TYPE ST_Control_UINT_TO_BIT :
STRUCT
	Enable_latch_C									:	BIT;
	Enable_latch_extern_on_positive_edge			:	BIT;
	Set_counter										:	BIT;
	Enable_latch_extern_on_negative_edge			:	BIT;
	{attribute 'hide'}
	reserve_b5										:	BIT;
	{attribute 'hide'}
	reserve_b6										:	BIT;
	{attribute 'hide'}
	reserve_b7										:	BIT;
	Set_counter_on_latch_C							:	BIT;
	
	Set_software_gate								:	BIT;
	Set_counter_on_latch_extern_on_positive_edge	:	BIT;
	Set_counter_on_latch_extern_on_negative_edge	:	BIT;
	Enable_latch_extern_2_on_positive_edge			:	BIT;
	Enable_latch_extern_2_on_negative_edge			:	BIT;
	{attribute 'hide'}
	reserve_b14										:	BIT;
	{attribute 'hide'}
	reserve_b15										:	BIT;
	{attribute 'hide'}
	reserve_b16										:	BIT;
END_STRUCT
END_TYPE
